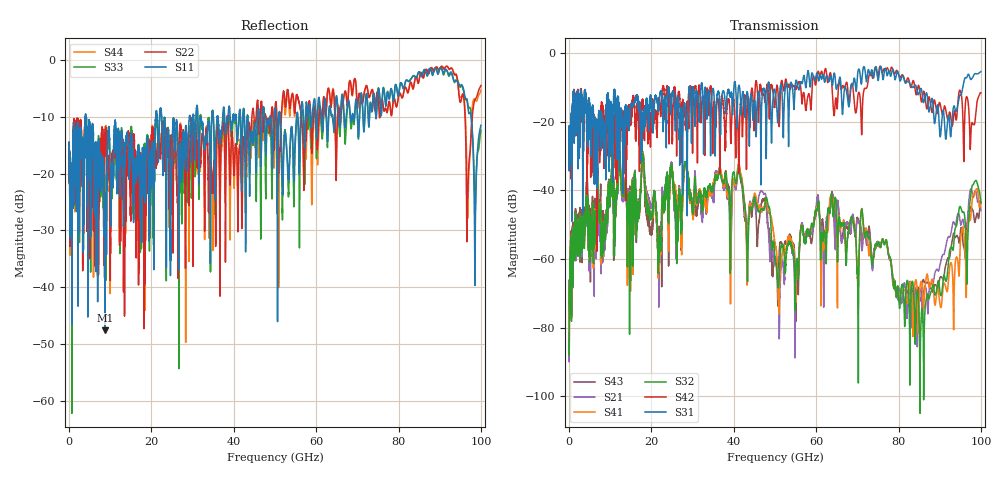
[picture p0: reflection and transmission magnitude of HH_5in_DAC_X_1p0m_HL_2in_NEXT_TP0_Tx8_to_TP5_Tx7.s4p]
# GHz S RI R 45
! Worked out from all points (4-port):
!   4000 points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, 25 MHz to 100 GHz, reference 45 ohm
!   strongest paths, dB at 25 MHz, 25.02 GHz, 50.02 GHz, 75.03 GHz, 100 GHz:
!     S31: -21.9, -11.6, -11.3, -7.9, -5.3
!     S42: -22.0, -22.6, -14.7, -7.0, -11.5
!     S32: -83.5, -33.5, -60.2, -55.4, -43.6
!     S41: -83.5, -33.4, -55.9, -55.1, -43.4
!     S21: -85.2, -33.4, -61.0, -55.2, -45.9
!     S43: -81.6, -33.3, -60.7, -55.1, -43.7
!   lowest |S11| = -47.5 dB at 8.75 GHz (marker M1), VSWR 1.01, Z = 45.2 + j0.329 ohm
!   |S11| at or under -10 dB: start of sweep to 4.02 GHz; 4.129 GHz to 21.05 GHz (16.92 GHz wide, 134 % of centre); 22.49 GHz to 29.27 GHz (6.781 GHz wide, 26.2 % of centre)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
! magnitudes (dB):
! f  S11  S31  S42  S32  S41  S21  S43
! 25 MHz  -15.6  -21.9  -22.0  -83.5  -83.5  -85.2  -81.6
! 8.75 GHz  -47.5  -22.8  -18.6  -48.2  -48.4  -48.4  -48.3
! 41.3 GHz  -9.9  -9.4  -27.0  -33.1  -32.3  -33.0  -32.8
! 51.02 GHz  -9.4  -13.7  -21.4  -65.7  -70.3  -78.3  -57.7
! 63.77 GHz  -9.9  -7.8  -8.3  -41.3  -42.5  -41.8  -40.8
! 85.75 GHz  -2.9  -11.9  -13.5  -74.4  -67.8  -77.3  -67.8
! 100 GHz  -11.5  -5.3  -11.5  -43.6  -43.4  -45.9  -43.7
